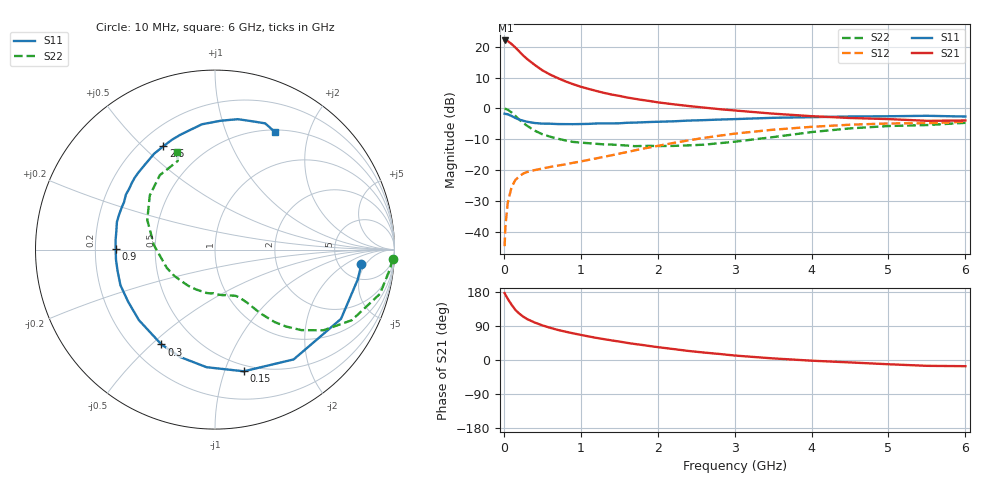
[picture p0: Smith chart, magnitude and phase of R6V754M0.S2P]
! SIEMENS Small Signal Semiconductors
! BFR193
! Si NPN RF Bipolar Junction Transistor in SOT23
! VCE = 0.75 V  IC = 4 mA
! Common Emitter S-Parameters:  May  1996
# GHz  S  MA  R  50
!  f  S11  S21  S12  S22
! GHz  MAG  ANG  MAG  ANG  MAG  ANG  MAG  ANG
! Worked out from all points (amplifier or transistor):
!   36 points, 10 MHz to 6 GHz, reference 50 ohm
!   highest |S21| = 22.0 dB at 20 MHz (marker M1)
!   |S21| within 3 dB of that: start of sweep to 177.9 MHz
!   unconditionally stable (mu >= 1): 917.4 MHz to 2.268 GHz
!   at 250 MHz: K = 0.38, MSG = 19.2 dB, |S12| = -21.2 dB
!   at 1.4 GHz: K = 1.10, MAG = 7.9 dB, |S12| = -15.3 dB
!   at 6 GHz: K = 1.00, MSG = 0.2 dB, |S12| = -4.3 dB
!   S11 on the Smith chart (normalised r, x): 10 MHz: 8.02, -4.04; 150 MHz: 0.44, -1.16; 300 MHz: 0.32, -0.54; 900 MHz: 0.29, +0.00; 2.6 GHz: 0.29, +0.58; 6 GHz: 0.52, +1.50
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0.01  0.8195 -5.8  12.58 176.6  0.0058 86.8  0.9904 -3.0
0.02  0.8126 -11.8  12.63 172.4  0.012 82.5  0.9815 -6.1
0.05  0.8012 -28.8  12.38 161.7  0.0291 75.1  0.9519 -15.0
0.1  0.7525 -54.4  11.06 146.0  0.0524 63.7  0.8576 -27.3
0.15  0.6967 -76.7  9.703 132.2  0.0688 54.4  0.7524 -36.7
0.2  0.6569 -94.1  8.384 122.5  0.079 48.7  0.6577 -43.0
0.25  0.6291 -108.0  7.221 114.7  0.0872 44.4  0.5828 -47.3
0.3  0.6068 -119.5  6.361 108.3  0.0924 42.0  0.5241 -50.5
0.4  0.5781 -137.1  5.078 99.0  0.0994 39.9  0.4348 -54.6
0.5  0.5645 -148.9  4.147 91.4  0.1055 39.3  0.3803 -56.9
0.6  0.563 -159.4  3.537 85.1  0.1119 39.6  0.3472 -58.7
0.7  0.5558 -167.5  3.101 79.5  0.1174 41.0  0.3218 -60.8
0.9  0.5534 179.8  2.466 70.4  0.1305 44.1  0.2853 -65.2
1.1  0.5592 169.3  2.068 62.3  0.1455 46.8  0.2719 -70.5
1.3  0.5688 159.9  1.785 55.1  0.1634 49.0  0.2603 -76.5
1.6  0.5832 148.3  1.501 45.3  0.1951 51.2  0.2489 -87.9
2.2  0.6154 128.7  1.165 29.0  0.2738 49.7  0.2457 -115.3
2.6  0.6436 116.6  1.029 19.7  0.3313 45.7  0.2571 -137.2
3.5  0.7019 96.0  0.82 4.2  0.4498 31.8  0.3413 175.8
4.5  0.7376 80.1  0.697 -6.4  0.5425 15.3  0.4727 140.2
5.5  0.7569 68.3  0.627 -15.4  0.5734 -0.4  0.5355 112.8
6  0.7358 63.2  0.636 -16.3  0.6062 -5.0  0.5816 111.2
